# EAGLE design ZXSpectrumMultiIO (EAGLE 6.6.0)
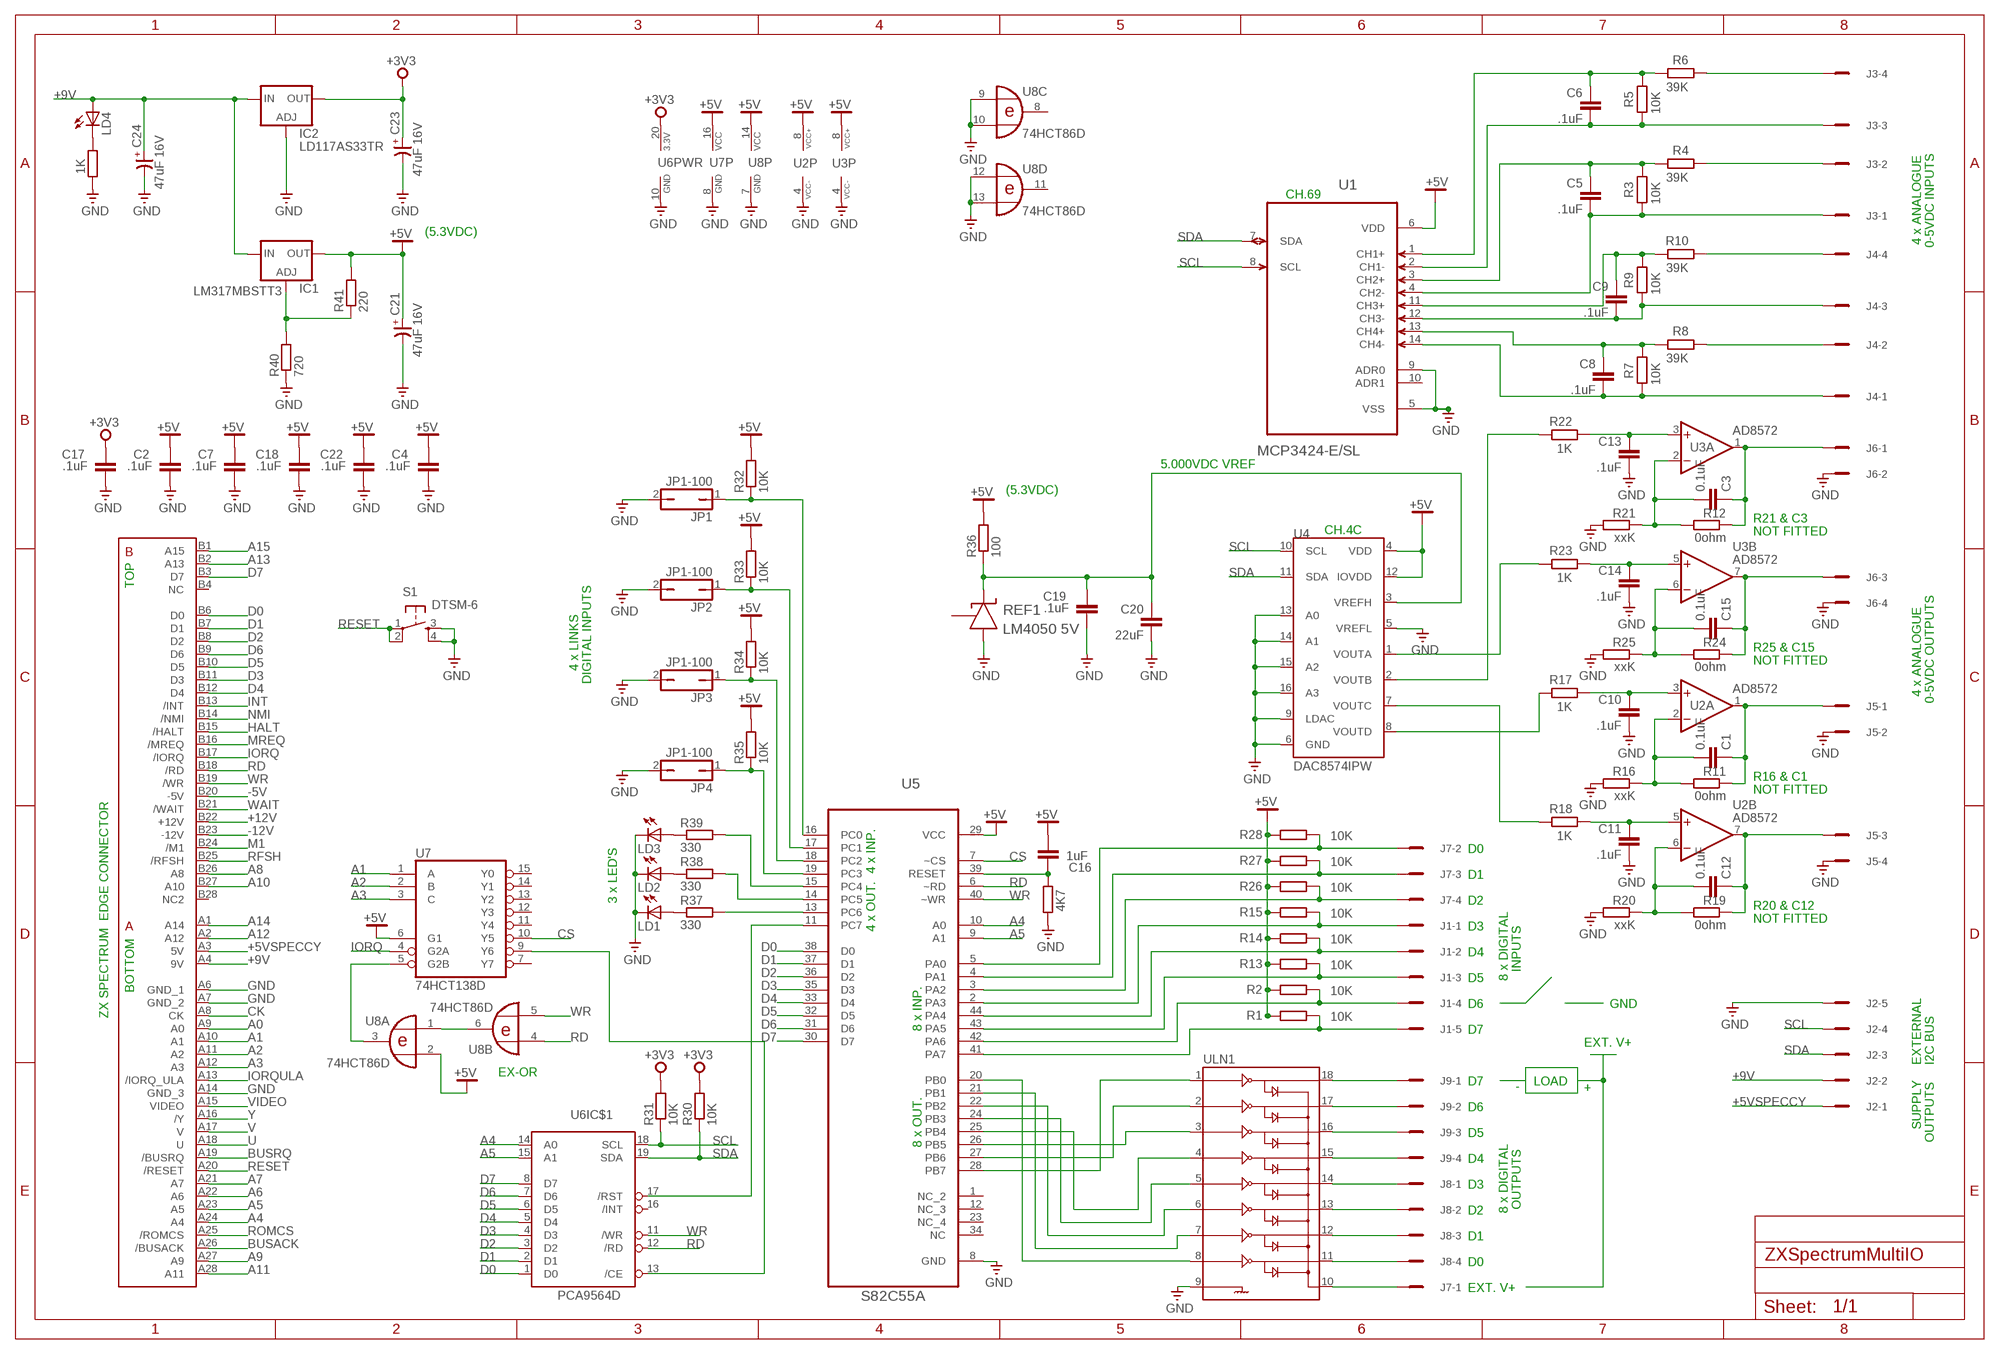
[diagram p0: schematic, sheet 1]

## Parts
C1  0.1uF  C-EUC0805  [C0805]
C2  .1uF  C-EUC0805  [C0805]
C3  0.1uF  C-EUC0805  [C0805]
C4  .1uF  C-EUC0805  [C0805]
C5  .1uF  C-EUC0805  [C0805]
C6  .1uF  C-EUC0805  [C0805]
C7  .1uF  C-EUC0805  [C0805]
C8  .1uF  C-EUC0805  [C0805]
C9  .1uF  C-EUC0805  [C0805]
C10  .1uF  C-EUC0805  [C0805]
C11  .1uF  C-EUC0805  [C0805]
C12  0.1uF  C-EUC0805  [C0805]
C13  .1uF  C-EUC0805  [C0805]
C14  .1uF  C-EUC0805  [C0805]
C15  0.1uF  C-EUC0805  [C0805]
C16  1uF  C-EUC0805  [C0805]
C17  .1uF  C-EUC0805  [C0805]
C18  .1uF  C-EUC0805  [C0805]
C19  .1uF  C-EUC0805  [C0805]
C20  22uF  C-EUC0805  [C0805]
C21  47uF 16V  CP-SV-C  [SV-C]
C22  .1uF  C-EUC0805  [C0805]
C23  47uF 16V  CP-SV-A  [SV-A]
C24  47uF 16V  CP-SV-C  [SV-C]
IC1  LM317MBSTT3  [SOT223]
IC2  LD117AS33TR  [SOT223]
J1  MCV5  [MCV5]
J2  MCV5  [MCV5]
J3  MCV4  [MCV4]
J4  MCV4  [MCV4]
J5  MCV4  [MCV4]
J6  MCV4  [MCV4]
J7  MCV4  [MCV4]
J8  MCV4  [MCV4]
J9  MCV4  [MCV4]
JP1  JP1-100  [JP1-100]
JP2  JP1-100  [JP1-100]
JP3  JP1-100  [JP1-100]
JP4  JP1-100  [JP1-100]
LD1  LEDCHIPLED_1206  [CHIPLED_1206]
LD2  LEDCHIPLED_1206  [CHIPLED_1206]
LD3  LEDCHIPLED_1206  [CHIPLED_1206]
LD4  LEDCHIPLED_1206  [CHIPLED_1206]
R1  10K  R-EU_R0805  [R0805]
R2  10K  R-EU_R0805  [R0805]
R3  10K  R-EU_R0805  [R0805]
R4  39K  R-EU_R0805  [R0805]
R5  10K  R-EU_R0805  [R0805]
R6  39K  R-EU_R0805  [R0805]
R7  10K  R-EU_R0805  [R0805]
R8  39K  R-EU_R0805  [R0805]
R9  10K  R-EU_R0805  [R0805]
R10  39K  R-EU_R0805  [R0805]
R11  0ohm  R-EU_R0805  [R0805]
R12  0ohm  R-EU_R0805  [R0805]
R13  10K  R-EU_R0805  [R0805]
R14  10K  R-EU_R0805  [R0805]
R15  10K  R-EU_R0805  [R0805]
R16  xxK  R-EU_R0805  [R0805]
R17  1K  R-EU_R0805  [R0805]
R18  1K  R-EU_R0805  [R0805]
R19  0ohm  R-EU_R0805  [R0805]
R20  xxK  R-EU_R0805  [R0805]
R21  xxK  R-EU_R0805  [R0805]
R22  1K  R-EU_R0805  [R0805]
R23  1K  R-EU_R0805  [R0805]
R24  0ohm  R-EU_R0805  [R0805]
R25  xxK  R-EU_R0805  [R0805]
R26  10K  R-EU_R0805  [R0805]
R27  10K  R-EU_R0805  [R0805]
R28  10K  R-EU_R0805  [R0805]
R29  4K7  R-EU_R0805  [R0805]
R30  10K  R-EU_R0805  [R0805]
R31  10K  R-EU_R0805  [R0805]
R32  10K  R-EU_R0805  [R0805]
R33  10K  R-EU_R0805  [R0805]
R34  10K  R-EU_R0805  [R0805]
R35  10K  R-EU_R0805  [R0805]
R36  100  R-EU_R0805  [R0805]
R37  330  R-EU_R0805  [R0805]
R38  330  R-EU_R0805  [R0805]
R39  330  R-EU_R0805  [R0805]
R40  720  R-EU_R0805  [R0805]
R41  220  R-EU_R0805  [R0805]
R42  1K  R-EU_R0805  [R0805]
REF1  LM4050 5V  LM4040A20IDBZT  [SOT95P237X112-3N]
S1  DTSM-6  [DTSM-6]
U1  MCP3424-E/SL  [SOIC127P600X175-14N]
U2  AD8572  TL072N  [SO08]
U3  AD8572  TL072N  [SO08]
U4  DAC8574IPW  [TSSOP16]
U5  S82C55A  CS82C55AZ  [PLCC127P1752X1752X457-44N]
U6  PCA9564D  [SO20W]
U7  74HCT138D  [SO16]
U8  74HCT86D  [SO14]
U$1  ZXSP_ED2X28_SPE_SOL_EDGE  [2X28_SPE2]
ULN1  ULN2803SOICW  [SO18L]

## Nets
+3V3: C17.1 C23.+ IC2.4(OUT) R30.2 R31.2 U6.20(PWR:3.3V)
+5V: C2.1 C4.1 C7.1 C16.2 C18.1 C21.+ C22.1 IC1.4(OUT) R1.2 R2.2 R13.2 R14.2 R15.2 R26.2 R27.2 R28.2 R32.2 R33.2 R34.2 R35.2 R36.2 R41.2 U1.6(VDD) U2.8(P:VCC+) U3.8(P:VCC+) U4.4(VDD) U4.12(IOVDD) U5.29(VCC) U7.6(G1) U7.16(VCC) U8.2(A:I1) U8.14(P:VCC)
+5VSPECCY: J2.1 U$1.A3(5V)
+9V: C24.+ IC1.3(IN) IC2.3(IN) J2.2 LD4.A U$1.A4(9V)
+12V: U$1.B22(+12V)
-5V: U$1.B20(-5V)
-12V: U$1.B23(-12V)
A0: U$1.A9(A0)
A1: U7.1(A) U$1.A10(A1)
A2: U7.2(B) U$1.A11(A2)
A3: U7.3(C) U$1.A12(A3)
A4: U5.10(A0) U6.14(IC$1:A0) U$1.A24(A4)
A5: U5.9(A1) U6.15(IC$1:A1) U$1.A23(A5)
A6: U$1.A22(A6)
A7: U$1.A21(A7)
A8: U$1.B26(A8)
A9: U$1.A27(A9)
A10: U$1.B27(A10)
A11: U$1.A28(A11)
A12: U$1.A2(A12)
A13: U$1.B2(A13)
A14: U$1.A1(A14)
A15: U$1.B1(A15)
BUSACK: U$1.A26(/BUSACK)
BUSRQ: U$1.A19(/BUSRQ)
CK: U$1.A8(CK)
CS: U5.7(~CS) U7.10(Y5)
D0: U5.38(D0) U6.1(IC$1:D0) U$1.B6(D0)
D1: U5.37(D1) U6.2(IC$1:D1) U$1.B7(D1)
D2: U5.36(D2) U6.3(IC$1:D2) U$1.B8(D2)
D3: U5.35(D3) U6.4(IC$1:D3) U$1.B11(D3)
D4: U5.33(D4) U6.5(IC$1:D4) U$1.B12(D4)
D5: U5.32(D5) U6.6(IC$1:D5) U$1.B10(D5)
D6: U5.31(D6) U6.7(IC$1:D6) U$1.B9(D6)
D7: U5.30(D7) U6.8(IC$1:D7) U$1.B3(D7)
GND: C2.2 C4.2 C7.2 C10.2 C11.2 C13.2 C14.2 C17.2 C18.2 C19.2 C20.2 C21.- C22.2 C23.- C24.- IC2.1(ADJ) J2.5 J5.2 J5.4 J6.2 J6.4 JP1.2 JP2.2 JP3.2 JP4.2 LD1.C LD2.C LD3.C R16.2 R20.2 R21.2 R25.2 R29.2 R40.1 R42.1 REF1.2(A) S1.3 S1.4 U1.5(VSS) U1.9(ADR0) U2.4(P:VCC-) U3.4(P:VCC-) U4.5(VREFL) U4.6(GND) U4.9(LDAC) U4.13(A0) U4.14(A1) U4.15(A2) U4.16(A3) U5.8(GND) U6.10(PWR:GND) U7.8(GND) U8.7(P:GND) U8.9(C:I0) U8.10(C:I1) U8.12(D:I0) U8.13(D:I1) U$1.A6(GND_1) U$1.A7(GND_2) U$1.A14(GND_3) ULN1.9
HALT: U$1.B15(/HALT)
INT: U$1.B13(/INT)
IORQ: U7.4(G2A) U$1.B17(/IORQ)
IORQULA: U$1.A13(/IORQ_ULA)
M1: U$1.B24(/M1)
MREQ: U$1.B16(/MREQ)
N$1: U5.20(PB0) ULN1.8
N$2: LD4.C R42.2
N$3: U7.5(G2B) U8.3(A:O)
N$4: U8.1(A:I0) U8.6(B:O)
N$5: R37.2 U5.13(PC6)
N$6: U5.21(PB1) ULN1.7
N$7: R38.2 U5.14(PC5)
N$8: R39.2 U5.15(PC4)
N$9: JP4.1 R35.1 U5.19(PC3)
N$10: JP3.1 R34.1 U5.18(PC2)
N$11: JP2.1 R33.1 U5.17(PC1)
N$12: JP1.1 R32.1 U5.16(PC0)
N$13: U5.22(PB2) ULN1.6
N$14: LD3.A R39.1
N$15: LD2.A R38.1
N$16: LD1.A R37.1
N$17: U6.13(IC$1:/CE) U7.9(Y6)
N$18: U5.11(PC7) U6.17(IC$1:/RST)
N$19: IC1.1(ADJ) R40.2 R41.1
N$21: C16.1 R29.1 U5.39(RESET)
N$22: U5.24(PB3) ULN1.5
N$23: U5.25(PB4) ULN1.4
N$24: U5.26(PB5) ULN1.3
N$25: U5.27(PB6) ULN1.2
N$26: U5.28(PB7) ULN1.1
N$30: C14.1 R23.1 U3.5(B:+IN)
N$31: C15.2 R24.2 R25.1 U3.6(B:-IN)
N$32: C15.1 J6.3 R24.1 U3.7(B:OUT)
N$33: C9.1 R9.1 R10.2 U1.11(CH3+)
N$34: C1.2 R11.2 R16.1 U2.2(A:-IN)
N$35: C10.1 R17.1 U2.3(A:+IN)
N$36: C11.1 R18.1 U2.5(B:+IN)
N$37: C12.2 R19.2 R20.1 U2.6(B:-IN)
N$38: C12.1 J5.3 R19.1 U2.7(B:OUT)
N$39: R22.2 U4.2(VOUTB)
N$40: R23.2 U4.1(VOUTA)
N$41: R18.2 U4.7(VOUTC)
N$42: R17.2 U4.8(VOUTD)
N$45: C19.1 C20.1 R36.1 REF1.1(CATHODE) U4.3(VREFH)
N$47: C5.2 J3.1 R3.2 U1.4(CH2-)
N$50: J4.2 R8.1
N$51: J4.4 R10.1
N$52: J3.2 R4.1
N$53: J3.4 R6.1
N$54: J1.5 R1.1 U5.41(PA7)
N$55: J1.4 R2.1 U5.42(PA6)
N$56: J9.1 ULN1.18
N$57: J9.2 ULN1.17
N$58: J9.3 ULN1.16
N$59: J9.4 ULN1.15
N$60: J8.1 ULN1.14
N$61: J8.2 ULN1.13
N$62: J8.3 ULN1.12
N$63: J8.4 ULN1.11
N$64: J7.1 ULN1.10
N$65: J1.3 R13.1 U5.43(PA5)
N$66: C3.2 R12.2 R21.1 U3.2(A:-IN)
N$67: C13.1 R22.1 U3.3(A:+IN)
N$68: J1.2 R14.1 U5.44(PA4)
N$69: J1.1 R15.1 U5.2(PA3)
N$70: J7.4 R26.1 U5.3(PA2)
N$71: J7.3 R27.1 U5.4(PA1)
N$72: J7.2 R28.1 U5.5(PA0)
N$78: C8.1 R7.1 R8.2 U1.13(CH4+)
N$79: C8.2 J4.1 R7.2 U1.14(CH4-)
N$80: C6.1 R5.1 R6.2 U1.1(CH1+)
N$81: C6.2 J3.3 R5.2 U1.2(CH1-)
N$82: C5.1 R3.1 R4.2 U1.3(CH2+)
N$83: C9.2 J4.3 R9.2 U1.12(CH3-)
NMI: U$1.B14(/NMI)
QQQ1: C3.1 J6.1 R12.1 U3.1(A:OUT)
QQQ2: C1.1 J5.1 R11.1 U2.1(A:OUT)
RD: U5.6(~RD) U6.12(IC$1:/RD) U8.4(B:I0) U$1.B18(/RD)
RESET: S1.1 S1.2 U$1.A20(/RESET)
RFSH: U$1.B25(/RFSH)
ROMCS: U$1.A25(/ROMCS)
SCL: J2.4 R31.1 U1.8(SCL) U4.10(SCL) U6.18(IC$1:SCL)
SDA: J2.3 R30.1 U1.7(SDA) U4.11(SDA) U6.19(IC$1:SDA)
U: U$1.A18(U)
V: U$1.A17(V)
VIDEO: U$1.A15(VIDEO)
WAIT: U$1.B21(/WAIT)
WR: U5.40(~WR) U6.11(IC$1:/WR) U8.5(B:I1) U$1.B19(/WR)
Y: U$1.A16(/Y)
Unconnected: REF1.3(NC) U1.10(ADR1) U5.1(NC_2) U5.12(NC_3) U5.23(NC_4) U5.34(NC) U6.16(IC$1:/INT) U7.7(Y7) U7.11(Y4) U7.12(Y3) U7.13(Y2) U7.14(Y1) U7.15(Y0) U8.8(C:O) U8.11(D:O) U$1.B4(NC) U$1.B28(NC2)

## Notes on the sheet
- CH.69
- (5.3VDC)
- 4 x ANALOGUE | 0-5VDC INPUTS
- 5.000VDC VREF
- (5.3VDC)
- R21 & C3
- CH.4C | NOT FITTED
- TOP
- R25 & C15
- NOT FITTED
- 4 x LINKS
- DIGITAL INPUTS
- 4 x ANALOGUE
- 0-5VDC OUTPUTS
- R16 & C1
- NOT FITTED
- D0
- 4 x INP.
- D1
- 3 x LED'S | D2
- R20 & C12
- NOT FITTED
- 4 x OUT. | D3
- D4
- INPUTS
- D5 | 8 x DIGITAL
- BOTTOM
- D6 | GND
- ZX SPECTRUM  EDGE CONNECTOR
- 8 x INP. | D7
- EXT. V+
- EXTERNAL | I2C BUS
- EX-OR
- 20L | 11 | D7 | LOAD
- - | +
- D6
- 1 | 10
- SUPPLY
- D5
- OUTPUTS
- 8 x OUT.
- D4
- D3
- OUTPUTS
- D2 | 8 x DIGITAL
- D1
- D0
- EXT. V+

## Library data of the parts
C1-C20 C22 = rcl:C-EU: CAPACITOR, European symbol
C21 C23 C24 = cap-master:CP-: POLARIZED CAP; PARTNO: *
IC1 = v-reg:LM317?*: 500 mA Adjustable Output Positive Voltage Regulator Source: http://www.onsemi.co.jp .. LM317M-D.PDF
IC2 = v-reg:LD117A?*: Low drop fixed and adjustable positive voltage regulators 1 A Source: http://www.st.com/stonline/products/literature/ds/7194/ld1117axx.pdf
J1 J2 = con-phoenix-381:MCV5: Mini-Combicon 3.81mm vertikal 5polig MCV 1,5/5-G-3,81 Artikel-Nr. 1803455
J3-J9 = con-phoenix-381:MCV4: Mini-Combicon 3.81mm vertikal 4polig MCV 1,5/4-G-3,81 Artikel-Nr. 1803442
JP1-JP4 = jumpers:JP1-: Jumper/Bridge
LD1-LD4 = led:LED: LED
R1-R42 = rcl:R-EU_: RESISTOR, European symbol
REF1 = LM4040:LM4040A20IDBZT: PRECISION MICROPOWER SHUNT VOLTAGE REFERENCE; MPN: LM4040A20IDBZT; OC_FARNELL: 1702826; OC_NEWARK: 53K9321; PACKAGE: 3-SOT-23; SUPPLIER: TEXAS INSTRUMENTS
S1 = switch-tact:DTSM-6
U1 = MCP3424:MCP3424-E/SL: Analog-to-Digital Converter; MPN: MCP3424-E/SL; OC_FARNELL: 1630424; OC_NEWARK: 54M4871; PACKAGE: SOIC-14; SUPPLIER: Microchip
U2 U3 = op-amp:TL072: JFET OP-AMP - Dual
U4 = DAC8574IPW:DAC8574IPW
U5 = 82C55:CS82C55AZ: CMOS Programmable Peripheral Interface; MPN: CS82C55AZ; OC_FARNELL: 9663533; OC_NEWARK: 42K8144; PACKAGE: PLCC-44; SUPPLIER: INTERSIL
U6 = i2c:PCA9564: Parallel Bus to I²C Bus Controller
U7 = 74xx-eu:74*138: 3-line to 8-line DECODER/DEMULTIPLEXER
U8 = 74xx-eu:74*86: Quad 2-input EXCLUSIVE-OR (XOR) gate
U$1 = zx_edge:ZXSP_ED
ULN1 = SparkFun-PowerIC:ULN2803: Darlington Driver ULN2803 Darlington array. 500mA max per channel, 8-channel package. Spark Fun Electronics SKU : COM-00312

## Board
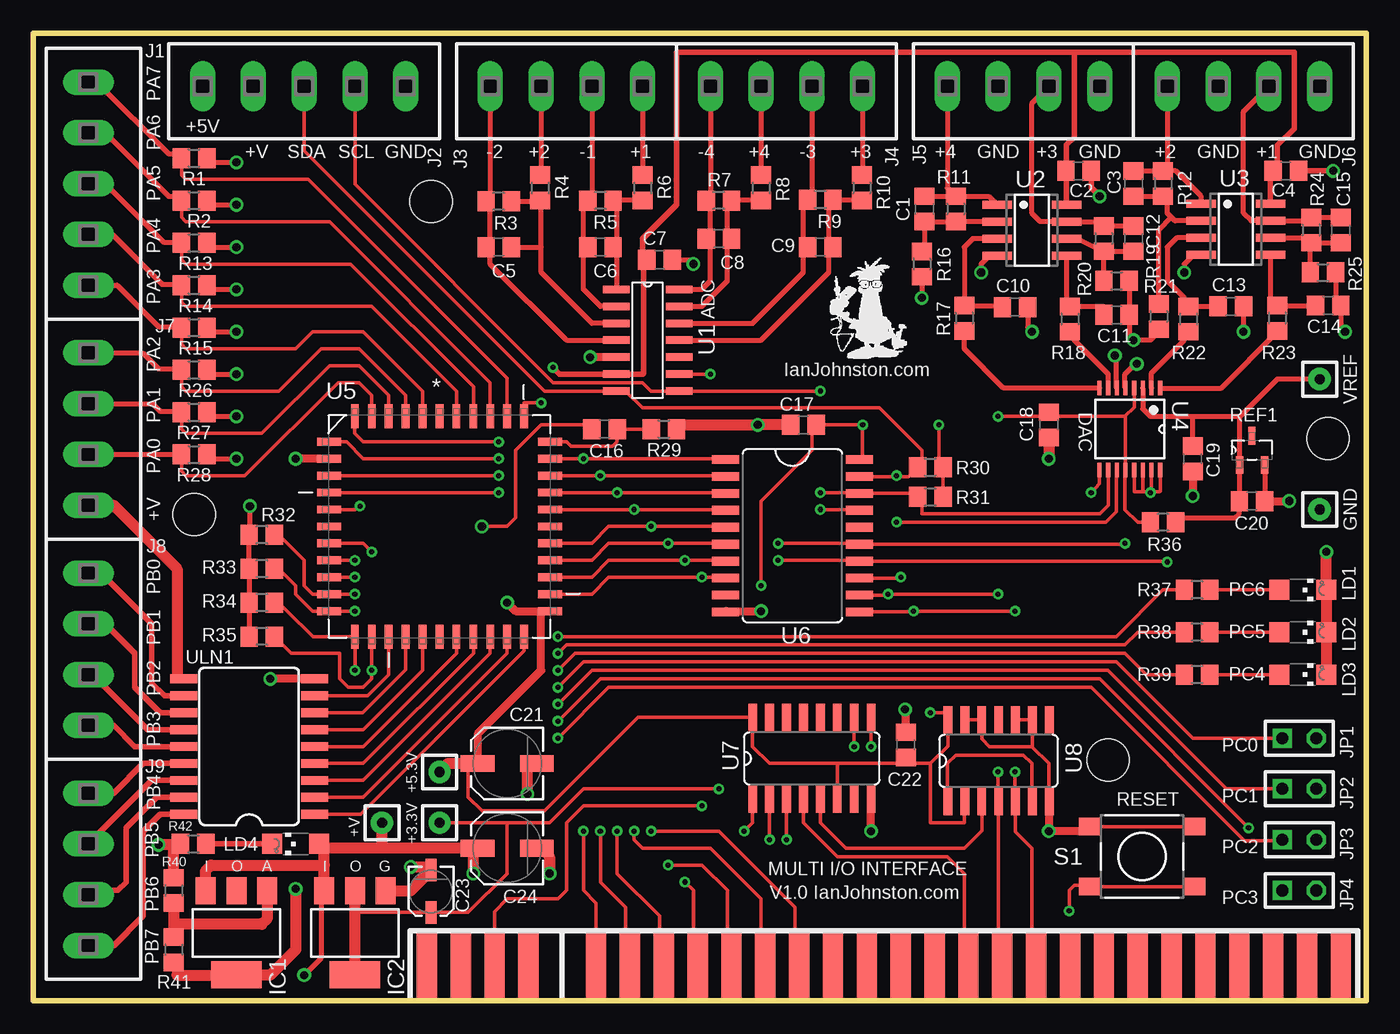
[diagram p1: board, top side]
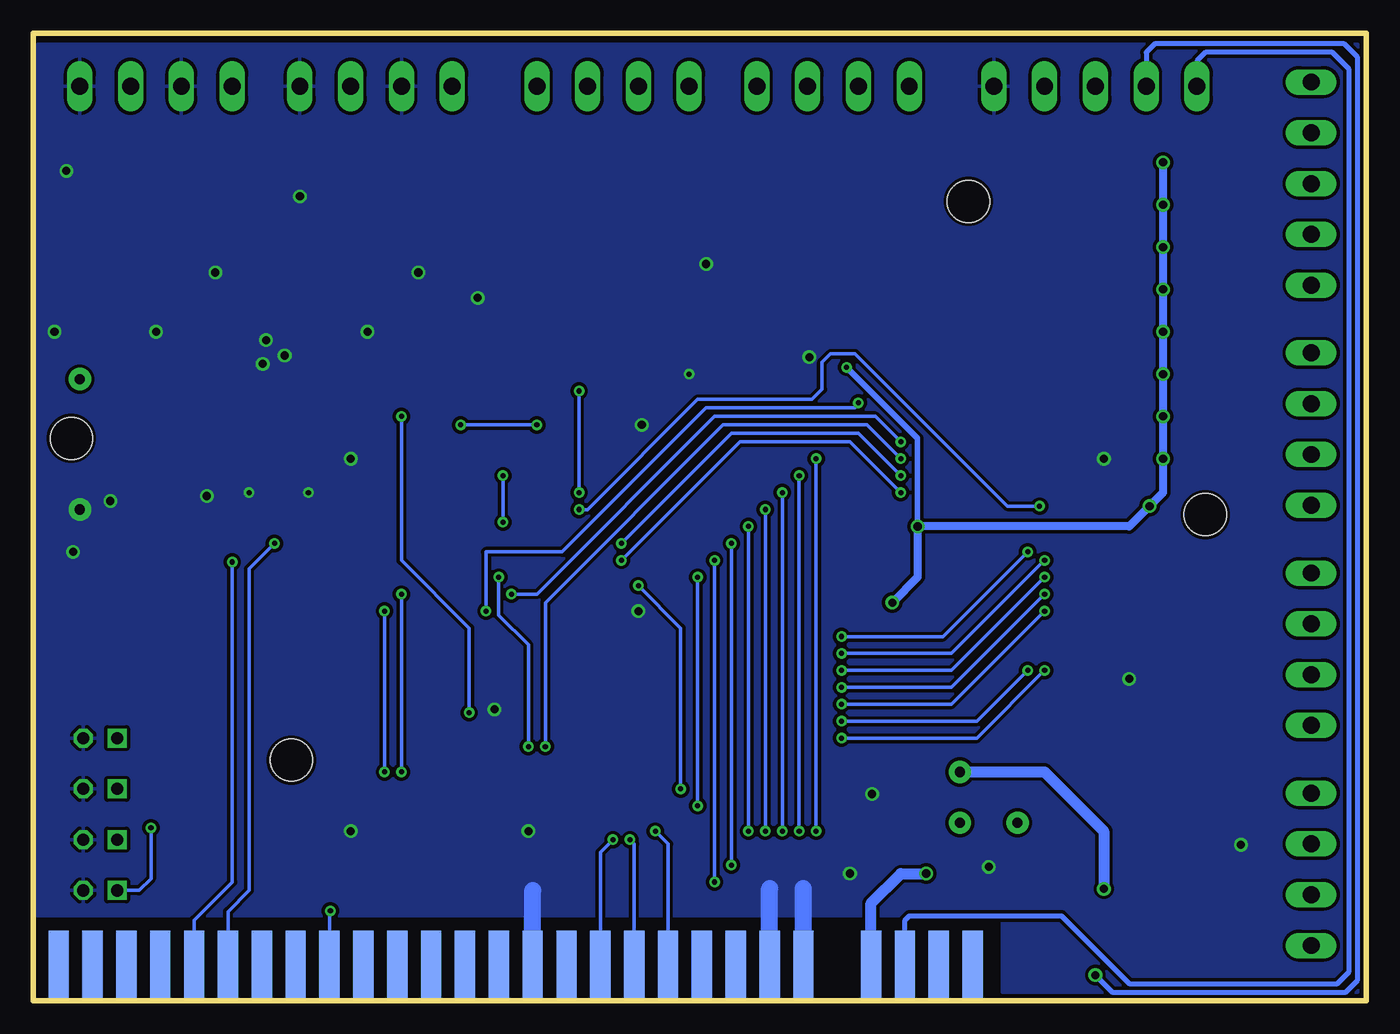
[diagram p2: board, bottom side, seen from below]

Size 100.01 x 72.55 mm. Coordinates in mm from the lower left corner, seen from the top.
Outline: 0,0 100.01,0 100.01,72.55 0,72.55 0,0
Copper layers (1*16): Top 0.035mm / dielectric 1.5mm / Bottom 0.035mm
Design rules "default": minimum track width 10mil, minimum drill 24mil, track to track 8mil, track to pad 8mil, pad to pad 8mil, via to via 8mil, smd to smd 8mil, copper to edge 0mil, drill to drill 8mil, minimum pad ring 10mil, minimum via ring 8mil, stop-mask expansion 4mil, vias tented up to drill 0mil, thermal gap 10mil
Holes 3.17 mm at 29.84,59.94 97.16,42.16 12.06,36.45 80.64,18.03

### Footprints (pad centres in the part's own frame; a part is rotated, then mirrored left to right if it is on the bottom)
C0805 = smd 1.3 x 1.5: 1 -0.95,0; 2 0.95,0
SV-C = smd 2.54 x 1.27: + -2.223,0; - 2.223,0
SV-A = smd 1.676 x 0.813: + -1.587,0; - 1.587,0
SOT223 = smd 1.5 x 2: 1 -2.3,-3.15; 2 0,-3.15; 3 2.3,-3.15 | smd 3.8 x 2: 4 0,3.15
MCV5 = drill 1.27 pad 1.905 long: 1 -7.62,0; 2 -3.81,0; 3 0,0; 4 3.81,0; 5 7.62,0
MCV4 = drill 1.27 pad 1.905 long: 1 -5.715,0; 2 -1.905,0; 3 1.905,0; 4 5.715,0
JP1-100 = drill 0.914 square: 1 0,-1.27 | drill 0.914 octagon: 2 0,1.27
CHIPLED_1206 = smd 1.5 x 1.5: A 0,-1.75; C 0,1.75
R0805 = smd 1.3 x 1.5: 1 -0.95,0; 2 0.95,0
SOT95P237X112-3N = smd 1.321 x 0.559: 1 -1.092,0.94; 2 -1.092,-0.94 | smd 1.321 x 0.508: 3 1.092,0
DTSM-6 = smd 1.55 x 1.3: 1 -3.975,2.25; 2 3.975,2.25; 3 -3.975,-2.25; 4 3.975,-2.25
SOIC127P600X175-14N = smd 1.981 x 0.559: 1 -2.362,3.81; 2 -2.362,2.54; 3 -2.362,1.27; 4 -2.362,0; 5 -2.362,-1.27; 6 -2.362,-2.54; 7 -2.362,-3.81; 8 2.362,-3.81; 9 2.362,-2.54; 10 2.362,-1.27; 11 2.362,0; 12 2.362,1.27; 13 2.362,2.54; 14 2.362,3.81
SO08 = smd 0.6 x 2.2: 1 -1.905,-2.6; 2 -0.635,-2.6; 3 0.635,-2.6; 4 1.905,-2.6; 5 1.905,2.6; 6 0.635,2.6; 7 -0.635,2.6; 8 -1.905,2.6
TSSOP16 = smd 0.31 x 1.1: 1 -2.275,-3.08; 2 -1.625,-3.08; 3 -0.975,-3.08; 4 -0.325,-3.08; 5 0.325,-3.08; 6 0.975,-3.08; 7 1.625,-3.08; 8 2.275,-3.08; 9 2.275,3.08; 10 1.625,3.08; 11 0.975,3.08; 12 0.325,3.08; 13 -0.325,3.08; 14 -0.975,3.08; 15 -1.625,3.08; 16 -2.275,3.08
PLCC127P1752X1752X457-44N = smd 0.584 x 1.803: 1 0,8.28; 2 -1.27,8.28; 3 -2.54,8.28; 4 -3.81,8.28; 5 -5.08,8.28; 6 -6.35,8.28; 18 -6.35,-8.28; 19 -5.08,-8.28; 20 -3.81,-8.28; 21 -2.54,-8.28; 22 -1.27,-8.28; 23 0,-8.28; 24 1.27,-8.28; 25 2.54,-8.28; 26 3.81,-8.28; 27 5.08,-8.28; 28 6.35,-8.28; 40 6.35,8.28; 41 5.08,8.28; 42 3.81,8.28; 43 2.54,8.28; 44 1.27,8.28 | smd 1.803 x 0.584: 7 -8.28,6.35; 8 -8.28,5.08; 9 -8.28,3.81; 10 -8.28,2.54; 11 -8.28,1.27; 12 -8.28,0; 13 -8.28,-1.27; 14 -8.28,-2.54; 15 -8.28,-3.81; 16 -8.28,-5.08; 17 -8.28,-6.35; 29 8.28,-6.35; 30 8.28,-5.08; 31 8.28,-3.81; 32 8.28,-2.54; 33 8.28,-1.27; 34 8.28,0; 35 8.28,1.27; 36 8.28,2.54; 37 8.28,3.81; 38 8.28,5.08; 39 8.28,6.35
SO20W = smd 0.66 x 2.032: 1 -5.715,-5.029; 2 -4.445,-5.029; 3 -3.175,-5.029; 4 -1.905,-5.029; 5 -0.635,-5.029; 6 0.635,-5.029; 7 1.905,-5.029; 8 3.175,-5.029; 9 4.445,-5.029; 10 5.715,-5.029; 11 5.715,5.029; 12 4.445,5.029; 13 3.175,5.029; 14 1.905,5.029; 15 0.635,5.029; 16 -0.635,5.029; 17 -1.905,5.029; 18 -3.175,5.029; 19 -4.445,5.029; 20 -5.715,5.029
SO16 = smd 0.66 x 2.032: 1 -4.445,-3.073; 2 -3.175,-3.073; 3 -1.905,-3.073; 4 -0.635,-3.073; 5 0.635,-3.073; 6 1.905,-3.073; 7 3.175,-3.073; 8 4.445,-3.073; 9 4.445,3.073; 10 3.175,3.073; 11 1.905,3.073; 12 0.635,3.073; 13 -0.635,3.073; 14 -1.905,3.073; 15 -3.175,3.073; 16 -4.445,3.073
SO14 = smd 0.66 x 2.032: 1 -3.81,-3.073; 2 -2.54,-3.073; 3 -1.27,-3.073; 4 0,-3.073; 5 1.27,-3.073; 6 2.54,-3.073; 7 3.81,-3.073; 8 3.81,3.073; 9 2.54,3.073; 10 1.27,3.073; 11 0,3.073; 12 -1.27,3.073; 13 -2.54,3.073; 14 -3.81,3.073
2X28_SPE2 = smd 1.524 x 5.08 bottom: A1 0,0; A2 2.54,0; A3 5.08,0; A4 7.62,0; A6 12.7,0; A7 15.24,0; A8 17.78,0; A9 20.32,0; A10 22.86,0; A11 25.4,0; A12 27.94,0; A13 30.48,0; A14 33.02,0; A15 35.56,0; A16 38.1,0; A17 40.64,0; A18 43.18,0; A19 45.72,0; A20 48.26,0; A21 50.8,0; A22 53.34,0; A23 55.88,0; A24 58.42,0; A25 60.96,0; A26 63.5,0; A27 66.04,0; A28 68.58,0 | smd 1.524 x 5.08: B1 0,0; B2 2.54,0; B3 5.08,0; B4 7.62,0; B6 12.7,0; B7 15.24,0; B8 17.78,0; B9 20.32,0; B10 22.86,0; B11 25.4,0; B12 27.94,0; B13 30.48,0; B14 33.02,0; B15 35.56,0; B16 38.1,0; B17 40.64,0; B18 43.18,0; B19 45.72,0; B20 48.26,0; B21 50.8,0; B22 53.34,0; B23 55.88,0; B24 58.42,0; B25 60.96,0; B26 63.5,0; B27 66.04,0; B28 68.58,0
SO18L = smd 0.66 x 2.032: 1 -0.635,-4.902; 2 0.635,-4.902; 3 1.905,-4.902; 4 3.175,-4.902; 5 4.445,-4.902; 6 5.715,-4.902; 7 6.985,-4.902; 8 8.255,-4.902; 9 9.525,-4.902; 10 9.525,4.902; 11 8.255,4.902; 12 6.985,4.902; 13 5.715,4.902; 14 4.445,4.902; 15 3.175,4.902; 16 1.905,4.902; 17 0.635,4.902; 18 -0.635,4.902

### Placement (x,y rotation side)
C1  66.87,59.37 270 top
C2  78.42,62.23 0 top
C3  82.55,61.28 270 top
C4  93.98,62.23 0 top
C5  34.92,56.52 180 top
C6  42.55,56.52 180 top
C7  46.99,55.56 0 top
C8  51.44,57.15 180 top
C9  59.05,56.52 180 top
C10  73.66,52.01 0 top
C11  81.28,51.44 0 top
C12  82.55,57.15 270 top
C13  89.85,52.07 0 top
C14  97.16,52.13 0 top
C15  98.11,57.78 270 top
C16  42.86,42.86 180 top
C17  57.78,43.18 180 top
C18  76.2,43.18 270 top
C19  87,40.64 270 top
C20  91.44,37.47 0 top
C21  35.56,17.78 0 top
C22  65.47,19.18 90 top
C23  29.84,8.19 90 top
C24  35.56,11.43 0 top
IC1  15.24,5.08 180 top
IC2  24.13,5.08 180 top
J1  4.13,61.28 90 top
J2  20.32,68.58 0 top
J3  40.01,68.58 0 top
J4  56.52,68.58 0 top
J5  74.3,68.58 0 top
J6  90.81,68.58 0 top
J7  4.13,42.86 90 top
J8  4.13,26.35 90 top
J9  4.13,9.84 90 top
JP1  95,19.68 270 top
JP2  95,15.88 270 top
JP3  95,12.06 270 top
JP4  95,8.26 270 top
LD1  95.25,30.8 270 top
LD2  95.25,27.62 270 top
LD3  95.25,24.45 270 top
LD4  19.68,11.75 90 top
R1  12.06,63.18 0 top
R2  12.06,60.01 0 top
R3  34.92,59.94 180 top
R4  38.04,60.96 270 top
R5  42.55,60.01 180 top
R6  45.72,60.96 270 top
R7  51.44,60.01 180 top
R8  54.61,60.96 270 top
R9  59.05,60.07 180 top
R10  62.17,60.96 270 top
R11  69.22,59.37 270 top
R12  84.77,61.28 270 top
R13  12.06,56.83 0 top
R14  12.06,53.66 0 top
R15  12.06,50.48 0 top
R16  66.67,55.24 270 top
R17  69.85,51.18 270 top
R18  77.79,51.12 270 top
R19  80.33,57.15 270 top
R20  81.28,53.98 0 top
R21  84.45,51.31 270 top
R22  86.68,51.12 270 top
R23  93.34,51.18 270 top
R24  95.89,57.78 270 top
R25  96.77,54.61 0 top
R26  12.06,47.31 0 top
R27  12.06,44.13 0 top
R28  12.06,40.96 0 top
R29  47.31,42.86 0 top
R30  67.31,40.01 0 top
R31  67.31,37.78 0 top
R32  17.14,34.92 180 top
R33  17.14,32.38 180 top
R34  17.14,29.84 180 top
R35  17.14,27.3 180 top
R36  84.77,35.88 180 top
R37  87.31,30.8 180 top
R38  87.31,27.62 180 top
R39  87.31,24.45 180 top
R40  10.54,8.26 270 top
R41  10.54,3.81 270 top
R42  12,11.75 0 top
REF1  91.44,41.27 90 top
S1  83.19,10.79 180 top
U1  46.1,49.53 0 top
U2  74.93,57.78 270 top
U3  90.23,57.85 270 top
U4  82.28,42.86 180 top
U5  30.48,35.56 0 top
U6  56.96,34.86 270 top
U7  58.42,18.16 0 top
U8  72.43,17.98 0 top
U$1  29.53,2.7 0 top
ULN1  16.19,14.61 90 top

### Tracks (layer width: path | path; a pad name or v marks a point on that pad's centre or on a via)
+3V3  (via drill 0.38, 0.76 pad 1.68)
  Top 0.254: U6.20 62.17,40.58 62.23,40.64 v62.23,43.18 C17.1 58.42,42.87 58.42,41.27 54.61,37.47 v54.61,31.11 | R31.2 R30.2 67.94,40.32 v67.94,43.18 | v51.44,15.88 41.27,15.88 38.73,13.34 35.56,13.34 | 35.56,13.34 35.56,9.53 32.64,6.6 C23.+ 24.13,6.6 IC2.4 | 35.56,13.34 v30.48,13.34
  Bottom 0.254: v67.94,43.18 v62.23,43.18 | v54.61,31.11 51.44,27.94 v51.44,15.88
+5V  (via drill 0.38, 0.61, 0.76 pad 1.68)
  Top 0.254: C7.1 45.78,55.5 45.78,55.31 45.72,55.24 | 81.92,43.81 76.52,43.81 C18.1 76.2,43.81 v72.39,43.81 | 81.92,43.81 81.95,43.78 U4.12 81.92,39.75 81.92,36.83 82.87,35.88 R36.2 | 32.64,17.78 32.64,17.72 | U7.6 60.33,17.78 | 60.33,17.78 55.24,17.78 53.98,19.05 U7.16 45.36,21.23 38.35,14.22 33.66,14.22 32.64,15.24 32.64,17.72 | 67.31,17.78 68.62,19.09 U8.14 68.58,21.1 68.58,21.59 v67.31,21.59 | 67.31,17.78 65.41,17.78 | 65.41,17.78 60.33,17.78 | U8.2 69.85,14.87 69.85,13.34 67.31,13.34 67.31,17.78 | C16.2 41.59,43.18 38.1,43.18 36.2,41.27 36.2,36.2 35.56,35.56 v33.66,35.56 | R32.2 16.26,34.99 | C22.1 65.41,18.16 65.41,17.78 | U4.4 82.6,44.5 81.92,43.81 | 32.64,17.72 C21.+ | R1.2 13.33,62.87 | R2.2 13.33,59.69 | R13.2 13.33,56.52 | R14.2 13.33,53.34 | R15.2 13.33,50.16 | R26.2 13.33,46.99 | R27.2 13.33,43.81 | R28.2 13.33,40.64
  Top 0.381: R32.2 R33.2 R34.2 R35.2 | 16.26,34.99 v16.26,37.08 | 13.33,62.87 v15.24,62.87 | 13.33,40.64 v15.24,40.64 | 13.33,56.52 v15.24,56.52 | 13.33,59.69 v15.24,59.69 | 13.33,53.34 v15.24,53.34 | 13.33,50.16 v15.24,50.16 | 13.33,46.99 v15.24,46.99 | 13.33,43.81 v15.24,43.81
  Top 0.406: 38.1,29.19 U5.29 | 45.78,55.5 45.78,47.05 45.72,46.99 U1.6 39.5,46.99 v38.99,47.5 | U2.8 77.53,62.17 | 77.53,62.17 C2.1 | U3.8 92.83,62.03 C4.1 93.34,62.55 93.34,64.14 94.61,65.41 94.61,71.12 78.11,71.12 | 77.53,62.17 77.53,64.19 78.11,64.77 78.11,71.12 | 78.11,71.12 48.26,71.12 48.26,59.69 45.72,57.15 45.72,55.24
  Top 0.61: 38.1,29.19 38.1,24.77 33.34,20 C21.+ | v35.56,29.84 36.2,29.21 U5.29
  Top 0.813: 32.64,17.78 C21.+ 31.11,17.78 v30.48,17.14 | R41.2 10.79,2.54 10.79,1.91 15.21,1.91 IC1.4 15.27,1.91 17.78,1.91 19.68,3.81 v19.68,8.38
  Bottom 0.254: v67.31,21.59 67.31,27.94 72.39,33.02 v72.39,43.81
  Bottom 0.406: v38.99,47.5 33.66,42.16 v33.66,35.56
  Bottom 0.61: v35.56,29.84 33.66,31.75 v33.66,35.56 17.78,35.56 v16.26,37.08 15.24,38.1 v15.24,40.64 v15.24,43.81 v15.24,46.99 v15.24,50.16 v15.24,53.34 v15.24,56.52 v15.24,59.69 v15.24,62.87
  Bottom 0.813: v30.48,17.14 24.13,17.14 19.68,12.7 v19.68,8.38
+5VSPECCY
  Bottom 0.381: U$1.A3 34.61,6.03 34.29,6.35 22.86,6.35 17.78,1.27 2.16,1.27 1.27,2.16 1.27,69.85 2.54,71.12 12.06,71.12 12.7,70.48 J2.1
+9V  (via drill 0.61, 0.76 pad 1.68)
  Top 0.381: v20.32,1.91 21.59,3.17 21.59,8.26 21.83,8.26 IC2.3
  Top 0.406: 32.38,11.11 C24.+ 33.02,11.11
  Top 0.813: C24.+ 26.16,11.43 | 26.16,11.43 21.59,11.43 21.59,11.59 LD4.A | v33.02,9.53 33.02,11.11 | 21.2,11.51 LD4.A | IC2.3 21.83,10.16 | 21.83,10.16 21.83,11.35 LD4.A | 26.16,11.43 v26.16,13.34 | IC1.3 12.94,9.77 13.34,10.16 21.83,10.16
  Bottom 0.381: v20.32,1.91 19.05,0.64 1.52,0.64 0.64,1.52 0.64,70.74 1.65,71.75 15.88,71.75 16.51,71.12 J2.2
  Bottom 0.813: U$1.A4 37.15,7.3 34.92,9.53 v33.02,9.53
A1  (via drill 0.38)
  Top 0.254: v53.34,12.7 53.98,13.34 U7.1
  Bottom 0.254: U$1.A10 52.39,11.75 v53.34,12.7
A2  (via drill 0.38)
  Top 0.254: v55.24,12.06 U7.2
  Bottom 0.254: U$1.A11 54.93,11.75 v55.24,12.06
A3  (via drill 0.38)
  Top 0.254: v56.52,12.06 U7.3
  Bottom 0.254: U$1.A12 57.47,11.11 v56.52,12.06
A4  (via drill 0.38)
  Top 0.254: U5.10 v34.92,38.1 | v55.88,33.02 61.92,33.02 U6.14 84.9,32.96 v85.09,32.89
  Bottom 0.254: U$1.A24 87.95,6.03 85.09,8.89 v85.09,32.89 | v34.92,38.1 38.73,41.91 46.99,41.91 v55.88,33.02
A5  (via drill 0.38)
  Top 0.254: 81.85,34.23 U6.15 61.92,34.29 v55.88,34.29 | U5.9 v34.92,39.37
  Top 0.406: 81.85,34.23 v81.92,34.29
  Bottom 0.254: U$1.A23 85.41,6.67 83.82,8.26 83.82,32.38 v81.92,34.29 | v34.92,39.37 38.1,42.55 47.62,42.55 v55.88,34.29
CS  (via drill 0.38)
  Top 0.254: U7.10 v61.59,19.05 | v34.92,40.64 24.77,40.64 23.5,41.91 U5.7
  Bottom 0.254: v61.59,19.05 61.59,29.84 48.26,43.18 37.47,43.18 v34.92,40.64
D0  (via drill 0.38)
  Top 0.254: U5.38 v41.27,40.64 51.87,40.64 U6.1 | U$1.B6 42.23,7.3 41.27,8.26 v41.27,12.7
  Bottom 0.254: v41.27,40.64 v41.27,12.7
D1  (via drill 0.38)
  Top 0.254: v42.55,39.37 39.37,39.37 39.31,39.31 38.82,39.31 U5.37 v42.55,39.37 | v42.55,39.37 51.87,39.37 U6.2 | v42.55,12.7 42.55,8.89 44.45,6.99 44.45,3.02 U$1.B7
  Bottom 0.254: v42.55,39.37 v42.55,12.7
D2  (via drill 0.38)
  Top 0.254: v43.81,38.1 39.37,38.1 39.31,38.04 38.82,38.04 U5.36 v43.81,38.1 | v43.81,38.1 51.87,38.1 U6.3 | v43.81,12.7 43.81,9.53 46.99,6.35 46.99,3.02 U$1.B8
  Bottom 0.254: v43.81,38.1 v43.81,12.7
D3  (via drill 0.38)
  Top 0.254: 39.37,36.83 U5.35 38.82,36.77 39.37,36.77 39.37,36.83 | U6.4 51.87,36.83 v45.09,36.83 39.37,36.83 | v45.09,12.7 45.09,12.06 45.72,11.43 50.8,11.43 54.61,7.62 54.61,3.02 U$1.B11
  Bottom 0.254: v45.09,36.83 v45.09,12.7
D4  (via drill 0.38)
  Top 0.254: U5.33 41.91,34.29 43.18,35.56 v46.35,35.56 51.87,35.56 U6.5 | v46.35,12.7 51.44,12.7 57.15,6.99 57.15,3.02 U$1.B12
  Bottom 0.254: v46.35,35.56 v46.35,12.7
D5  (via drill 0.38)
  Top 0.254: U5.32 41.91,33.02 43.18,34.29 v47.62,34.29 51.87,34.29 U6.6 | v47.62,10.16 50.16,10.16 52.07,8.26 52.07,3.02 U$1.B10
  Bottom 0.254: v47.62,34.29 v47.62,10.16
D6  (via drill 0.38)
  Top 0.254: 52.07,33.02 52.01,32.96 U6.7 51.87,33.02 v48.9,33.02 43.18,33.02 41.91,31.75 U5.31 38.73,31.75 | v48.9,8.89 49.53,8.26 49.53,3.02 U$1.B9
  Bottom 0.254: v48.9,33.02 v48.9,8.89
D7  (via drill 0.38)
  Top 0.254: U5.30 41.91,30.48 43.18,31.75 v50.16,31.75 | v50.16,31.75 51.87,31.75 U6.8 51.93,31.75 v50.16,31.75 | U$1.B3 34.61,6.67 35.56,7.62 39.37,7.62 40.01,8.26 40.01,13.34 41.27,14.61 v50.16,14.61
  Bottom 0.254: v50.16,31.75 v50.16,14.61
GND  (via drill 0.38, 0.61, 0.76 pad 1.68)
  Top 0.254: U1.9 v50.8,46.99 | U4.9 80,38.74 v79.38,38.1 | U4.13 82.6,38.15 83.82,38.15 | U4.16 84.55,38.2 84.5,38.15 83.9,38.15 | U4.15 83.9,38.15 | U4.14 83.25,38.16 83.82,38.16 83.82,38.15 | U2.4 72.33,55.82 71.75,55.88 | U3.4 87.63,55.88 87,55.88 | U8.13 U8.12 71.16,19.64 71.75,19.05 74.93,19.05 74.97,19.01 | U8.10 U8.9 74.97,19.01 | 74.97,19.01 76.2,17.78 76.2,15.59 U8.7 | R29.2 48.58,43.18 | U6.10 51.99,29.21 | 83.82,38.15 v83.82,38.1 | 83.82,38.15 83.9,38.15 | S1.4 S1.3 79.03,13.04 | R21.2 84.45,50.16 | 97.72,52.51 C14.2 | REF1.2 | U4.5 81.92,45.98 | U4.6 81.28,45.96 | LD2.C 96.36,28.09 96.52,27.94 96.52,28.1 LD2.C
  Top 0.381: 71.75,55.88 71.12,55.24 v71.12,54.61 | 87,55.88 86.36,55.24 v86.36,54.61 | C10.2 74.61,50.48 v74.93,50.16 | C13.2 90.8,50.8 v90.81,50.16 | C14.2 98.11,50.48 v98.42,50.16 | C7.2 49.21,55.56 v49.53,55.24 | R16.2 v66.67,52.7 | R20.2 C11.2 82.23,49.85 v82.55,49.53 83.82,49.53 84.45,50.16 | R25.2 97.72,52.51 | REF1.2 C20.2 | 81.92,45.98 81.92,46.99 82.68,47.75 v82.8,47.75 | 81.28,45.96 81.28,48.26 v81.15,48.39
  Top 0.406: C2.2 79.37,60.96 v80.01,60.33 | C4.2 v97.54,62.23
  Top 0.61: U1.5 v41.78,48.26 | R42.1 10.93,11.43 | ULN1.9 v17.78,24.13 | U5.8 v19.68,40.64 | C22.2 65.47,21.78 v65.41,21.84 | 51.99,29.21 v54.61,29.21 | 79.03,13.04 78.74,12.7 v76.2,12.7 76.2,14.91 U8.7 | C20.2 v94.23,37.47 | v62.87,12.7 U7.8 | C19.2 v87,37.85
  Top 0.813: LD3.C LD2.C LD1.C 97,33.63 v97.03,33.66 | C18.2 v76.2,40.64 | v37.08,15.49 37.08,17.78 C21.- | C17.2 v54.36,43.18 48.58,43.18 | 10.54,11.68 11.05,11.68 10.8,11.43 10.93,11.43 | IC2.1 28.3,8.23 C23.- 29.34,10.03 v28.32,10.03 | C24.- 38.42,11.11 38.73,10.79 v38.73,9.53 | R40.1 10.54,11.68 | 10.54,11.68 v9.4,11.68
  Bottom 0.406: U$1.A7 44.77,2.54
  Bottom 1.27: U$1.A6 42.23,8.41 | 44.77,2.54 44.77,8.41 | U$1.A14 62.55,8.26
  other vias: 96.52,36.83
  pour Bottom (isolate 0.254): 0.64,71.73 0.64,0.61 27.3,0.61 27.3,6.35 99.69,6.33 99.69,71.73
IORQ
  Top 0.254: U7.4 57.78,13.34 60.33,10.79 68.58,10.79 69.85,9.53 69.85,3.02 U$1.B17
N$1
  Top 0.254: ULN1.8 25.08,22.86 26.67,24.45 U5.20
  Top 0.406: U5.20
N$2
  Top 0.406: LD4.C R42.2
N$3
  Top 0.254: U8.3 71.16,12.74 69.85,11.43 60.96,11.43 59.05,13.34 U7.5
N$4
  Top 0.254: U8.1 68.58,15.59 68.58,17.78 69.22,18.41 74.3,18.41 74.93,17.78 74.93,15.59 U8.6
N$5  (via drill 0.38)
  Top 0.254: R37.2 84.77,30.8 81.28,27.3 v39.37,27.3 | v25.4,33.66 24.77,34.29 U5.13
  Bottom 0.254: v39.37,27.3 31.75,27.3 v25.4,33.66
N$6
  Top 0.254: ULN1.7 24.7,21.59 27.94,24.83 U5.21
  Top 0.406: U5.21
N$7  (via drill 0.38)
  Top 0.254: R38.2 82.87,27.62 81.92,26.67 40.01,26.67 v39.37,26.04 | v24.13,33.02 U5.14
  Bottom 0.254: v39.37,26.04 31.11,26.04 v24.13,33.02
N$8  (via drill 0.38)
  Top 0.254: R39.2 83.5,24.45 81.92,26.04 40.64,26.04 v39.37,24.77 | v24.13,31.75 U5.15
  Bottom 0.254: v39.37,24.77 31.11,24.77 v24.13,31.75
N$9  (via drill 0.38)
  Top 0.254: v91.19,12.95 80.01,24.13 42.55,24.13 v39.37,20.95 | U5.19 v25.4,24.77 25.4,24.13 24.77,23.5 23.62,23.5 22.99,24.13 22.99,26.04 19.36,26.04 R35.1
  Bottom 0.254: v39.37,20.95 29.21,20.95 v25.4,24.77 | v91.19,12.95 91.19,9.14 92.08,8.26 JP4.1
N$10  (via drill 0.38)
  Top 0.254: v39.37,19.68 43.18,23.5 79.38,23.5 90.87,12 93.66,12 JP3.1 | v24.13,24.77 U5.18 20.98,27.28 19.05,29.21 18.41,29.84 R34.1
  Bottom 0.254: v39.37,19.68 29.21,19.68 v24.13,24.77
N$11  (via drill 0.38)
  Top 0.254: JP2.1 89.53,15.88 80.64,24.77 41.91,24.77 v39.37,22.23 | U5.17 v24.13,29.21 20.95,29.21 19.68,30.48 19.68,31.11 18.41,32.38 R33.1
  Bottom 0.254: v39.37,22.23 31.11,22.23 v24.13,29.21
N$12  (via drill 0.38)
  Top 0.254: JP1.1 87,19.68 81.28,25.4 41.27,25.4 v39.37,23.5 | U5.16 v24.13,30.48 20.95,30.48 20.32,31.11 20.32,33.02 18.41,34.92 R32.1
  Bottom 0.254: v39.37,23.5 31.11,23.5 v24.13,30.48
N$13
  Top 0.254: ULN1.6 24.77,20.32 29.21,24.77 U5.22
  Top 0.406: U5.22
N$14
  Top 0.254: R39.1 LD3.A
N$15
  Top 0.254: R38.1 LD2.A
N$16
  Top 0.254: R37.1 LD1.A
N$17  (via drill 0.38)
  Top 0.254: U7.9 v62.87,19.05 | v65.09,31.75 65.02,31.69 U6.13
  Bottom 0.254: v62.87,19.05 62.87,26.67 65.09,28.89 v65.09,31.75
N$18  (via drill 0.38)
  Top 0.254: U6.17 61.92,36.83 v59.05,36.83 | v24.51,37.08 24.38,37.08 24.13,36.83 U5.11
  Bottom 0.254: v59.05,36.83 58.42,36.83 50.16,45.09 41.59,45.09 40.83,45.85 40.83,47.88 40.2,48.51 38.35,48.51 26.92,37.08 v24.51,37.08
N$19
  Top 0.813: R40.2 10.54,5.71 | 10.54,5.71 R41.1 | IC1.1 17.54,6.11 17.14,5.71 10.54,5.71
N$20
  Top 0.813: 24.13,1.91 24.13,8.26
N$21
  Top 0.254: U5.39 40.01,41.91 40.35,41.56 43.47,41.56 43.81,41.91 C16.1 R29.1
N$22
  Top 0.254: ULN1.5 24.77,19.05 31.75,26.04 U5.24
  Top 0.406: U5.24
N$23
  Top 0.254: ULN1.4 24.77,17.78 33.02,26.04 U5.25
  Top 0.406: U5.25
N$24
  Top 0.254: ULN1.3 24.77,16.51 34.29,26.04 U5.26
  Top 0.406: U5.26
N$25
  Top 0.254: ULN1.2 24.77,15.24 35.56,26.04 U5.27
  Top 0.406: U5.27
N$26
  Top 0.254: ULN1.1 24.57,13.97 36.83,26.23 U5.28
  Top 0.406: U5.28
N$30
  Top 0.254: 92.83,52.64 R23.1 | C14.1
  Top 0.381: U3.5 92.83,52.64 | R23.1 C14.1
N$31
  Top 0.254: 95.51,57.21 R24.2 95.82,56.77
  Top 0.381: U3.6 95.51,57.21 | R24.2 C15.2 | R25.1 95.82,56.77
N$32
  Top 0.254: 95.63,58.48 R24.1
  Top 0.381: 95.63,58.48 U3.7 91.38,58.48 90.81,59.05 90.81,66.67 J6.3 | R24.1 C15.1
N$33
  Top 0.254: 60.07,60.01 R9.1 59.69,59.76 | C9.1 59.69,56.52
  Top 0.381: R10.2 60.07,60.01 | U1.11 54.61,49.53 59.69,54.61 59.69,56.52 59.69,59.76
N$34
  Top 0.254: R11.2 | 66.86,56.39 R16.1
  Top 0.381: U2.2 R11.2 | R11.2 C1.2 66.86,56.39
N$35
  Top 0.254: 72.58,52.13 C10.1
  Top 0.381: U2.3 70.48,57.15 69.85,56.52 R17.1 72.58,52.13
N$36
  Top 0.254: 77.53,52.33 R18.1 | 80.33,52.07 C11.1
  Top 0.381: U2.5 77.53,52.33 | R18.1 80.33,52.07
N$37
  Top 0.254: U2.6 78.36,57.15 | 79.63,56.52 80.01,55.88 R19.2
  Top 0.381: 78.36,57.15 79.63,56.52 | R19.2 C12.2 | R20.1 R19.2
N$38
  Top 0.254: 80.01,58.42 R19.1
  Top 0.381: 80.01,58.42 U2.7 75.56,58.42 74.93,59.05 74.93,67.31 J5.3 | R19.1 C12.1
N$39
  Top 0.254: 86.36,49.53 86.36,49.85 R22.2
  Top 0.381: U4.2 83.9,47.07 86.36,49.53
N$40
  Top 0.254: 93.34,50.16 R23.2
  Top 0.381: U4.1 89.12,45.94 93.34,50.16
N$41
  Top 0.254: 78.11,49.85 R18.2
  Top 0.381: U4.7 80.65,46.98 78.11,49.53 78.11,49.85
N$42
  Top 0.381: U4.8 72.8,45.94 69.85,48.9 R17.2
N$45  (via drill 0.76 pad 1.68)
  Top 0.254: REF1.1 | R36.1 86.04,36.2 | 90.55,43.81 90.5,43.76
  Top 0.381: v96.52,46.61 93.34,46.61 90.55,43.81 87,43.81 | U4.3 83.25,44.38 83.82,43.81 87,43.81 | REF1.1 C20.1 90.49,36.52 90.17,36.2 86.04,36.2 | 90.5,43.76 REF1.1 | C19.1 87,43.81
N$47
  Top 0.254: 34.29,60.26 R3.2 34.29,59.63 | C5.2 34.29,56.52
  Top 0.381: J3.1 34.29,60.26 | 34.29,59.63 34.29,56.52 34.29,55.24 40.01,49.53 U1.4
N$50
  Top 0.381: J4.2 R8.1
N$51
  Top 0.254: 62.23,61.97 R10.1
  Top 0.381: J4.4 62.23,61.97
N$52
  Top 0.254: 38.1,61.97 R4.1
  Top 0.381: J3.2 38.1,61.97
N$53
  Top 0.381: J3.4 R6.1
N$54
  Top 0.254: U5.41 35.56,46.67 20.64,61.59 11.43,61.59 11.12,61.91 R1.1
  Top 0.381: J1.5 4.76,68.9 10.16,63.5 10.8,63.5 R1.1
  Top 0.406: U5.41
N$55
  Top 0.254: U5.42 34.29,46.35 22.23,58.42 11.43,58.42 11.12,58.73 R2.1
  Top 0.381: J1.4 5.4,65.09 10.16,60.33 10.8,60.33 R2.1
  Top 0.406: U5.42
N$56
  Top 0.406: J9.1 6.03,4.13 8.26,6.35 8.26,12.7 9.53,13.97 ULN1.18
N$57
  Top 0.406: ULN1.17 9.27,15.24 6.99,12.95 6.99,8.89 6.35,8.26 4.45,8.26 J9.2
N$58
  Top 0.406: ULN1.16 8.89,16.51 J9.3
N$59
  Top 0.406: ULN1.15 8.26,17.78 6.03,15.56 J9.4
N$60
  Top 0.406: J8.1 6.03,20.64 7.62,19.05 ULN1.14
N$61
  Top 0.406: J8.2 4.45,24.45 8.57,20.32 ULN1.13
N$62
  Top 0.406: ULN1.12 9.53,21.59 7.62,23.5 7.62,26.04 5.4,28.26 J8.3
N$63
  Top 0.406: J8.4 5.08,32.07 8.89,28.26 8.89,23.81 9.84,22.86 ULN1.11
N$64
  Top 0.406: 10.79,24.27 ULN1.10
  Top 0.813: 10.79,24.27 10.79,32.38 6.03,37.15 J7.1
N$65
  Top 0.254: U5.43 33.02,46.04 23.81,55.24 11.43,55.24 11.12,55.56 R13.1 11.43,57.15
  Top 0.381: J1.3 5.4,61.28 9.78,56.9 11.05,56.9 R13.1
  Top 0.406: U5.43
N$66
  Top 0.254: 85.09,60.01 R12.2
  Top 0.381: C3.2 R12.2 | U3.2 85.66,58.48 85.41,58.74 | 85.41,58.74 85.09,59.05 85.09,60.01 | R21.1 84.45,57.78 85.41,58.74
N$67
  Top 0.254: 86.36,52.7 R22.1 | 88.27,52.07 C13.1
  Top 0.381: U3.3 85.79,57.21 85.09,56.52 85.09,53.98 86.36,52.7 | R22.1 88.27,52.07
N$68
  Top 0.254: U5.44 31.75,45.72 25.4,52.07 11.43,52.07 11.12,52.38 R14.1 10.8,53.98
  Top 0.381: J1.2 5.91,57.47 9.65,53.72 11.05,53.72 R14.1
  Top 0.406: U5.44
N$69
  Top 0.254: U5.2 29.21,45.72 24.77,50.16 20.95,50.16 19.68,48.9 11.43,48.9 11.12,49.21 R15.1 11.43,50.8
  Top 0.381: J1.1 6.29,53.66 9.4,50.55 11.05,50.55 R15.1
  Top 0.406: U5.2
N$70
  Top 0.254: U5.3 27.94,45.4 24.45,48.9 21.59,48.9 18.41,45.72 11.43,45.72 11.12,46.03 R26.1
  Top 0.381: J7.4 8.19,48.58 9.4,47.37 11.05,47.37 R26.1
  Top 0.406: U5.3
N$71
  Top 0.254: U5.4 26.67,45.4 24.45,47.62 22.23,47.62 17.14,42.55 11.43,42.55 11.12,42.86 R27.1
  Top 0.381: J7.3 8.95,44.77 9.53,44.2 11.05,44.2 R27.1
  Top 0.406: U5.4
N$72
  Top 0.254: U5.5 25.4,45.4 24.45,46.35 22.86,46.35 15.88,39.37 11.43,39.37 11.12,39.69 R28.1
  Top 0.381: J7.2 R28.1
  Top 0.406: U5.5
N$78
  Top 0.254: R7.1 52.07,59.69 | C8.1 52.07,57.15
  Top 0.381: R8.2 R7.1 | U1.13 50.16,52.07 52.07,53.98 52.07,57.15 52.07,59.69
N$79
  Top 0.254: 50.8,60.32 R7.2 50.8,59.69 | C8.2 50.8,57.15
  Top 0.381: J4.1 50.8,60.32 | U1.14 50.16,53.34 50.8,53.98 50.8,57.15 50.8,59.69
N$80
  Top 0.254: 43.74,59.76 R5.1 | U1.1 43.81,53.34 | 43.81,59.69 R5.1 | R5.1 | C6.1 43.81,56.52
  Top 0.381: 43.81,53.34 43.81,56.52 43.81,59.69 | R6.2 R5.1
N$81
  Top 0.254: 41.91,60.32 R5.2 41.27,59.69 | C6.2 41.27,56.52
  Top 0.381: J3.3 41.91,60.32 | U1.2 42.55,52.07 41.27,53.34 41.27,56.52 41.27,59.69
N$82
  Top 0.254: 37.97,59.94 R4.2 38.1,59.95
  Top 0.381: R3.1 37.97,59.94 | U1.3 41.91,50.8 38.1,54.61 38.1,56.52 | 38.1,56.52 38.1,59.95 | C5.1 38.1,56.52
N$83
  Top 0.254: 58.42,60.39 R9.2 57.78,59.75 | C9.2 57.78,56.52
  Top 0.381: J4.3 58.42,60.39 | U1.12 53.98,50.8 57.78,54.61 57.78,56.52 57.78,59.75
QQQ1
  Top 0.254: R12.1 85.09,62.55
  Top 0.381: C3.1 R12.1 | U3.1 87.63,60.32 85.72,62.23 R12.1 | J6.1 85.09,62.55
QQQ2
  Top 0.381: J5.1 68.58,60.96 R11.1 | C1.1 R11.1 | R11.1 71.7,60.32 U2.1
RD  (via drill 0.38)
  Top 0.254: U$1.B18 72.43,2.98 U8.4 72.39,14.95 v72.39,17.14 | U5.6 24.13,42.55 24.77,41.91 v34.92,41.91 | U6.12 64.07,30.42 v64.14,30.48 v72.39,30.48
  Bottom 0.254: v34.92,41.91 36.83,43.81 48.9,43.81 62.23,30.48 v64.14,30.48 | v72.39,17.14 v72.39,30.48
RESET  (via drill 0.38)
  Top 0.254: v77.72,6.73 77.72,8.26 78.11,8.64 78.99,8.64 S1.2 S1.1
  Bottom 0.254: U$1.A20 77.79,6.67 v77.72,6.73
SCL  (via drill 0.38)
  Top 0.254: v59.05,45.72 U1.8 46.35,45.72 45.72,46.35 38.99,46.35 24.13,61.21 J2.4 | v59.05,38.1 61.92,38.1 U6.18 66.11,38.04 R31.1 66.67,37.47 66.67,36.51 80.01,36.51 80.65,37.15 U4.10
  Bottom 0.254: v59.05,38.1 v59.05,45.72
SDA  (via drill 0.38)
  Top 0.254: U4.11 81.28,39.76 81.28,36.67 80.49,35.88 v64.77,35.88 | 64.77,39.31 65.66,39.31 R30.1 66.67,40.32 66.67,41.27 63.5,44.45 45.72,44.45 44.45,45.72 U1.7 38.35,45.72 20.32,63.75 J2.3 | U6.19 64.77,39.31 | 64.77,39.31 v64.77,39.37
  Bottom 0.254: v64.77,35.88 v64.77,39.37
WR  (via drill 0.38)
  Top 0.254: U$1.B19 74.93,3.02 74.93,11.43 73.7,12.66 U8.5 73.66,14.95 v73.66,17.14 | U5.40 36.85,43.84 36.85,44.04 36.83,44.83 v38.1,44.83 | U6.11 65.98,29.15 v66.04,29.21 v73.66,29.21
  Bottom 0.254: v38.1,44.83 38.35,44.45 49.53,44.45 60.33,33.66 66.04,33.66 v66.04,29.21 | v73.66,17.14 v73.66,29.21

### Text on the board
tNames: PA7 | +5V | PA6 | +V | SDA | SCL | GND | -2 | +2 | -1 | +1 | -4 | +4 | -3 | +3 | +4 | GND | +3 | GND | +2 | GND | +1 | GND | PA5 | PA4 | PA3 | ADC | PA2 | IanJohnston.com | VREF | DAC | PA1 | PA0 | +V | GND | PB0 | PC6 | PB1 | PC5 | PC4 | PB2 | PC0 | PB3 | +5.3V | PC1 | RESET | PB4 | +V | +3.3V | PC2 | PB5 | I | O | A | I | O | G | MULTI I/O INTERFACE | V1.0 IanJohnston.com | PC3 | PB6 | PB7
